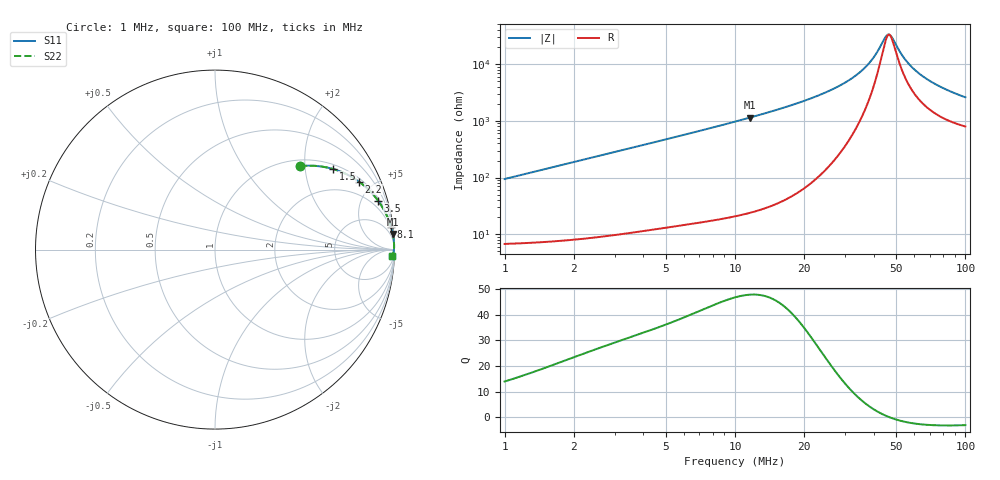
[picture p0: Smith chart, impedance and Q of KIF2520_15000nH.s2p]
!version-2
!date-12.2020
!Series
# MHz S RI R 50
!Freq ReS11 ImS11 ReS21 ImS21 ReS12 ImS12 ReS22 ImS22
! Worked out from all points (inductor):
!   991 points, 1 MHz to 100 MHz, reference 50 ohm
!   read as one part in series: L = 14.9 uH near 1.4 MHz
!   highest Q = 47.7 at 11.6 MHz (marker M1), where L = 15.7 uH
!   self-resonance near 46.7 MHz
!   S11 on the Smith chart (normalised r, x): 1 MHz: 1.14, +1.88; 1.5 MHz: 1.15, +2.82; 2.2 MHz: 1.17, +4.14; 3.5 MHz: 1.21, +6.58; 8.1 MHz: 1, +15; 100 MHz: 17, -49
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1  0.4731 0.4646  0.5269 -0.4646  0.5269 -0.4646  0.4731 0.4646
1.5  0.6586 0.4489  0.3414 -0.4489  0.3414 -0.4489  0.6586 0.4489
2.2  0.8012 0.3794  0.1988 -0.3794  0.1988 -0.3794  0.8012 0.3794
3.5  0.9081 0.2733  0.0919 -0.2733  0.0919 -0.2733  0.9081 0.2733
5.5  0.9596 0.1841  0.0404 -0.1841  0.0404 -0.1841  0.9596 0.1841
8.1  0.9807 0.1265  0.0193 -0.1265  0.0193 -0.1265  0.9807 0.1265
11.6  0.9906 0.0866  0.00941 -0.0866  0.00941 -0.0866  0.9906 0.0866
17.5  0.9959 0.053  0.00412 -0.053  0.00412 -0.053  0.9959 0.053
28.5  0.9979 0.0238  0.00209 -0.0238  0.00209 -0.0238  0.9979 0.0238
34  0.9979 0.0149  0.00209 -0.0149  0.00209 -0.0149  0.9979 0.0149
39.3  0.9976 0.008  0.00235 -0.008  0.00235 -0.008  0.9976 0.008
44.6  0.9972 0.00215  0.00279 -0.00215  0.00279 -0.00215  0.9972 0.00215
45.8  0.9971 0.00093  0.00291 -0.00093  0.00291 -0.00093  0.9971 0.00093
47.5  0.9969 -0.000734  0.00309 0.000734  0.00309 0.000734  0.9969 -0.000734
50.5  0.9966 -0.00352  0.00344 0.00352  0.00344 0.00352  0.9966 -0.00352
53.6  0.9962 -0.00623  0.00383 0.00623  0.00383 0.00623  0.9962 -0.00623
57.2  0.9957 -0.00919  0.00434 0.00919  0.00434 0.00919  0.9957 -0.00919
61.6  0.995 -0.0126  0.00501 0.0126  0.00501 0.0126  0.995 -0.0126
67  0.9941 -0.0165  0.00591 0.0165  0.00591 0.0165  0.9941 -0.0165
74.4  0.9927 -0.0214  0.00727 0.0214  0.00727 0.0214  0.9927 -0.0214
83.5  0.9909 -0.0269  0.00913 0.0269  0.00913 0.0269  0.9909 -0.0269
100  0.9871 -0.0357  0.0129 0.0357  0.0129 0.0357  0.9871 -0.0357
